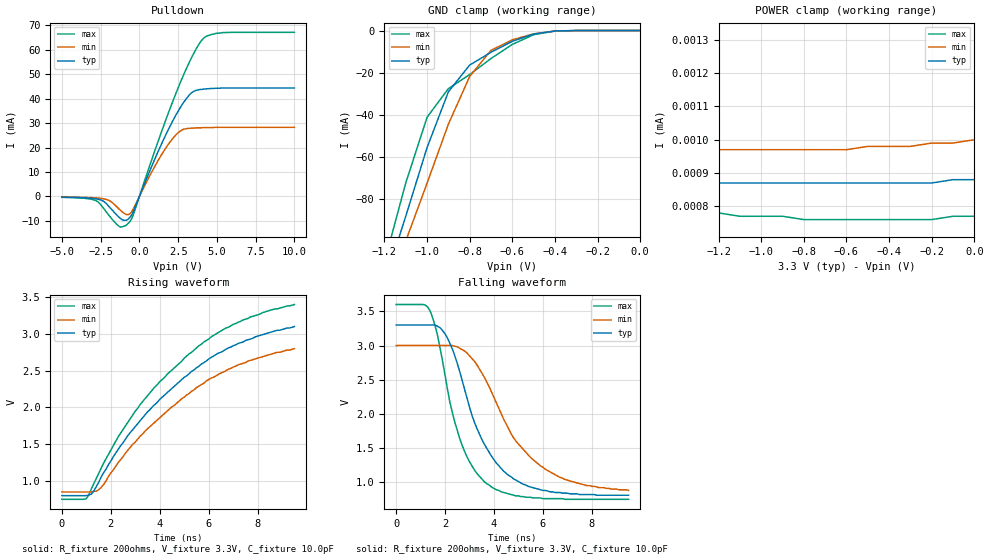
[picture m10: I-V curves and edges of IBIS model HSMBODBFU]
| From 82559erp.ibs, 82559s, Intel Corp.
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[Model]   HSMBODBFU
Model_type   I/O_open_drain
Vinl  =   0.6
Vinh  =   1.4
|   typ   min   max
C_comp   2.2pF   NA   NA
| note : on die power/gnd supply distribution R/L/C
|   are not included in the simulation
| note : pull up  mos are not active  pup#="1"
| note : POWER_clamp ref = VIO = VREF = 5.0V
| variable   typ   min   max
[Voltage range]   3.3V   3.0V   3.6V
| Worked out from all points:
|   slope of the pulldown table from 0 to 0.495 V, typ, clamps not added: 63.8 ohm
|   GND clamp passes 1 mA (typ) near -0.45 V on its own axis
|   POWER clamp passes 1 mA (typ) near -2.33 V on its own axis
|   rising waveform, R_fixture 200ohms, V_fixture 3.3V, C_fixture 10.0pF: 20-80 % time 3.95ns typ, 3.92ns min, 3.97ns max; typ from 0.8 V to 3.1 V
|   falling waveform, R_fixture 200ohms, V_fixture 3.3V, C_fixture 10.0pF: 20-80 % time 1.6ns typ, 2.15ns min, 1.21ns max; typ from 3.3 V to 0.81 V
| note : all DC curves are with 0.2 OHM res. in series to the PAD.
[GND_clamp]
|Voltage   I(typ)   I(min)   I(max)
-5V       -1.63A     -1.47A     -1.85A
-1.2V     -120mA     -130mA     -110mA
-1.1V     -88.2mA    -100mA     -72.4mA
-1V       -55.6mA    -72.5mA    -41.2mA
-900mV    -29.1mA    -44.5mA    -27.6mA
-800mV    -16.4mA    -21.8mA    -20.9mA
-700mV    -10.3mA    -9.4mA     -13.3mA
-600mV    -5.12mA    -4.42mA    -6.6mA
-500mV    -1.67mA    -1.57mA    -2mA
-400mV    -240uA     -300uA     -220uA
0V        0A         0A         0A
[PullDown]
| Voltage   I(typ)   I(min)   I(max)
-5V       -320uA     -230uA     -400uA
-2.8V     -1.01mA    -630uA     -1.76mA
-2.2V     -2.55mA    -1.14mA    -5.84mA
-1.4V     -8mA       -4.64mA    -11.8mA
-900mV    -9.77mA    -7.25mA    -12mA
-400mV    -6.32mA    -5.21mA    -7.64mA
1.2V      18.3mA     14.7mA     22.4mA
2.2V      31.5mA     24.1mA     39.7mA
3.3V      42.1mA     27.9mA     56mA
4V        43.8mA     28.1mA     63.8mA
5.4V      44.4mA     28.3mA     67.1mA
10V       44.4mA     28.3mA     67.2mA
[POWER_clamp]
| Voltage   I(typ)   I(min)   I(max)
-5V       11.7A      10.4A      13A
-2.4V     3.43mA     4.33uA     460mA
-2.3V     100uA      1.19uA     140mA
-2.2V     3.74uA     1.04uA     9.93mA
-2.1V     1.02uA     1.03uA     170uA
-2V       930nA      1.02uA     3.25uA
-1.9V     920nA      1.01uA     860nA
-1.8V     910nA      1uA        820nA
-1.2V     870nA      970nA      780nA
-800mV    870nA      970nA      760nA
-300mV    870nA      980nA      760nA
0V        880nA      1uA        770nA
[Ramp]   | note : pad parasitics are not included
|Variable   typ   min   max
dV/dt_r   1.5/2.0n   1.3/2.1n   1.7/2.0n
dV/dt_f   1.5/9.5n   1.3/13.5n   1.7/6.5n
| note : 200ohms RES. always connected to VCC
R_load =   200ohms
[Rising Waveform]
| note : pad parasitics are not included
| note : input changes at T=0.5nS
| note : input data is to vox_data
R_fixture   = 200ohms
V_fixture   = 3.3V
V_fixture_min   = 3.0V
V_fixture_max   = 3.6V
C_fixture   = 10.0pF
| note : the 200ohms RES. is connected to VCC
|Time   typ   min   max
0s        800mV      850mV      750mV
1ns       800mV      850mV      760mV
1.3ns     860mV      860mV      960mV
1.6ns     1.05V      910mV      1.17V
2.3ns     1.43V      1.25V      1.6V
3ns       1.74V      1.53V      1.95V
3.8ns     2.04V      1.8V       2.28V
5.2ns     2.46V      2.19V      2.73V
7ns       2.84V      2.55V      3.13V
9.5ns     3.1V       2.8V       3.4V
[Falling Waveform]
| note : pad parasitics are not included
| note : input changes at T=0.5nS
| note : input data is to vox_data
R_fixture   = 200ohms
V_fixture   = 3.3V
V_fixture_min   = 3.0V
V_fixture_max   = 3.6V
C_fixture   = 10.0pF
| note : the 200ohms RES. is connected to VCC
|Time   typ   min   max
0s        3.3V       3V         3.6V
1.4ns     3.3V       3V         3.5V
1.7ns     3.28V      3V         3.14V
2ns       3.17V      3V         2.57V
2.6ns     2.62V      2.96V      1.64V
3.1ns     1.98V      2.81V      1.24V
3.7ns     1.5V       2.47V      980mV
4.8ns     1.05V      1.65V      810mV
5.9ns     890mV      1.24V      770mV
9.5ns     810mV      880mV      750mV
